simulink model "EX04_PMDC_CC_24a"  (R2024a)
settings: Solver=ode45  StartTime=0.0  StopTime=0.2  MaxStep=1e-5  RelTol=1e-3  EnableMultiTasking=on
undefined symbols (not defined in the file): A, constant, N, Torque
libraries: spsControlledVoltageSourceLib x1, spsCurrentMeasurementLib x1, spsDCMachineLib x1, spspowerguiLib x1

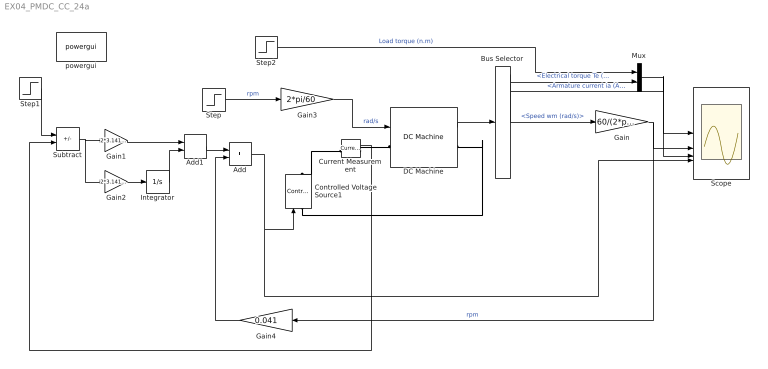
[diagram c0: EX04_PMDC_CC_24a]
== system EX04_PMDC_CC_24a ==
  Add : Sum
  Add1 : Sum
  Bus Selector : BusSelector  OutputSignals=Electrical torque Te (n m),Speed wm (rad/s),Armature current ia (A)
  Controlled Voltage Source1 : spsControlledVoltageSourceLib/Controlled Voltage Source  Initialize=on  Source_Type=AC  Amplitude=0  Phase=0  Frequency=0  Measurements=Voltage
  Current Measurement : spsCurrentMeasurementLib/Current Measurement  PhasorSimulation=off  OutputType=Complex  PSBequivalent=0
  DC Machine : spsDCMachineLib/DC Machine  PresetModel=No  MechanicalLoad=Speed w  FieldType=Permanent magnet  ShowDetailedParameters=on  MeasurementBus=off  RLa=[0.26 1.7e-3]  RLf="[ 240  120]"  Laf=1.8  MachineConstant=Torque constant (N.m/A)  Ke=0.04415  Kt=0.3937  J=0.00252  Bm=0  Tf=0  w0=0  Ifinit=1  TsPowergui=0  TsBlock=-1
  Gain : Gain  Gain=60/(2*pi)
  Gain1 : Gain  Gain=2*3.141592*300*1.7e-3
  Gain2 : Gain  Gain=2*3.141592*300*0.26
  Gain3 : Gain  Gain=2*pi/60
  Gain4 : Gain  Gain=0.041
  Integrator : Integrator
  Mux : Mux  Inputs=2
  Scope : Scope  NumInputPorts=4
  Step : Step  Time=0.15  After=3000  SampleTime=0
  Step1 : Step  Time=0.1  After=24.9  SampleTime=0
  Step2 : Step  Time=0.1  After=9.8039  SampleTime=0
  Subtract : Sum  Inputs=+-
  powergui : spspowerguiLib/powergui  Priority=1  SimulationMode=Continuous  SampleTime=50e-6  frequency=60  Iterations=50  frequencyindice=0  Pbase=100e6  ErrMax=1e-4  UnitsV=kV  UnitsW=MW  buscounter=0  FunctionMessages=off  echomessages=off  EnableUseOfTLC=off  CurrentSourceSwitches=off  DisableSnubberDevices=on  DisableRonSwitches=on  DisableVfSwitches=on  DisplayEquations=off  AutomaticDiscreteSolvers=off  SolverType=Tustin  Interpol=off  ExternalGateDelay=off  methode=off  Ts=0  x0status=blocks  SPID=on  SwTol=0  HookPort=off  NonlinearTolerance=1e-4  nMaxIteration=100  ContinueOnMaxIteration=off  RestoreLinks=warning  ResistiveCurrentMeasurement=off  Frange=[0:2:500]  Ylog=off  Xlog=on  ShowGrid=off  save=off  variable=ZData  structure=0  ZoomFFT=off  StartTime=0.0  cycles=1  DisplayStyle=1  fundamental=60  FreqAxis=off  MaxFrequency=1000  frequencyindicesteady=1  RmsSteady=1  display=off
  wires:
  DC Machine/1 -> Bus Selector/1
  Bus Selector/2 -> Gain/1  "<Speed wm (rad/s)>"
  Bus Selector/3 -> Scope/3  "<Armature current ia (A)>"
  Gain/1 -> Gain4/1, Scope/2  "rpm"
  Step2/1 -> Mux/1  "Load torque (n.m)"
  Mux/1 -> Scope/1
  Bus Selector/1 -> Mux/2  "<Electrical torque Te (n m)>"
  Step/1 -> Gain3/1  "rpm"
  Current Measurement/1 -> Subtract/2
  Step1/1 -> Subtract/1
  Subtract/1 -> Gain2/1, Gain1/1
  Gain2/1 -> Integrator/1
  Add/1 -> Scope/4, Controlled Voltage Source1/1
  Gain3/1 -> DC Machine/1  "rad/s"
  Add1/1 -> Add/1
  Integrator/1 -> Add1/2
  Gain1/1 -> Add1/1
  Gain4/1 -> Add/2
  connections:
  Controlled Voltage Source1/LConn1 -- DC Machine/RConn1
  Current Measurement/RConn1 -- DC Machine/LConn1
  Current Measurement/LConn1 -- Controlled Voltage Source1/RConn1
